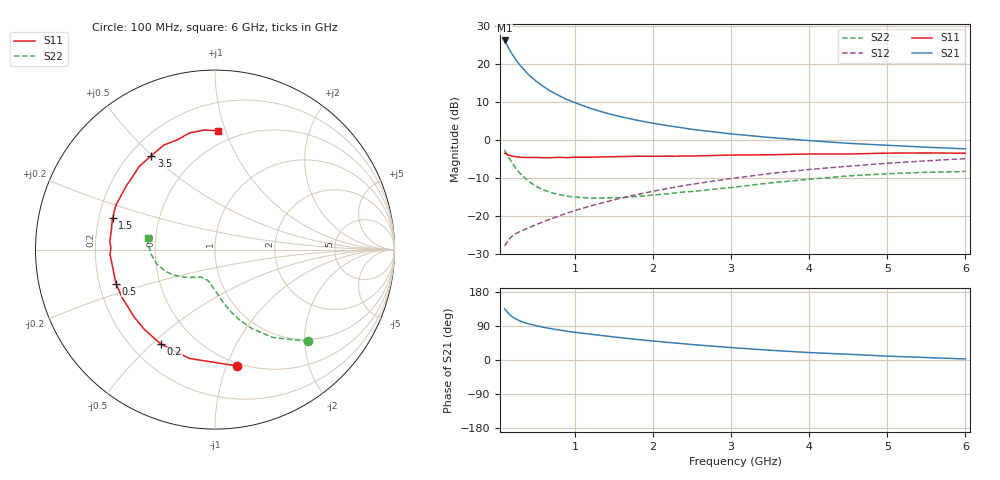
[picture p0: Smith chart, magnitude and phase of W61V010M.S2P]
! SIEMENS Small Signal Semiconductors
! BFR193W
! Si NPN RF Bipolar Junction Transistor in SOT323
! VCE = 1 V  IC = 10 mA
! Common Emitter S-Parameters:  September  1992
# GHz  S  MA  R  50
!  f  S11  S21  S12  S22
! GHz  MAG  ANG  MAG  ANG  MAG  ANG  MAG  ANG
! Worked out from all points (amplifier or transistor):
!   28 points, 100 MHz to 6 GHz, reference 50 ohm
!   highest |S21| = 26.1 dB at 100 MHz (marker M1)
!   |S21| within 3 dB of that: start of sweep to 179.9 MHz
!   unconditionally stable (mu >= 1): 892.4 MHz to 2.755 GHz
!   at 300 MHz: K = 0.57, MSG = 21.8 dB, |S12| = -24.1 dB
!   at 1.5 GHz: K = 1.06, MAG = 9.6 dB, |S12| = -15.8 dB
!   at 6 GHz: K = 0.95, MSG = 1.3 dB, |S12| = -5.0 dB
!   S11 on the Smith chart (normalised r, x): 100 MHz: 0.47, -1.09; 200 MHz: 0.32, -0.54; 500 MHz: 0.27, -0.15; 1.5 GHz: 0.26, +0.14; 3.5 GHz: 0.28, +0.50; 6 GHz: 0.40, +0.94
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0.1  0.6596 -79.3  20.18 135.3  0.0397 56.4  0.7291 -44.5
0.15  0.623 -103.2  16.11 122.6  0.0484 49.7  0.5863 -56.6
0.2  0.6067 -119.7  13.18 113.8  0.0542 46.5  0.4854 -65.0
0.25  0.5937 -131.6  11.02 107.7  0.0585 45.4  0.4094 -71.2
0.3  0.5867 -140.0  9.453 102.9  0.0622 45.5  0.3584 -75.6
0.4  0.5827 -152.8  7.275 95.8  0.0687 46.9  0.2868 -82.3
0.5  0.5831 -161.1  5.913 90.7  0.0759 49.3  0.2441 -87.2
0.6  0.5785 -167.7  4.975 86.3  0.0836 51.2  0.2178 -91.9
0.7  0.5798 -172.8  4.277 82.5  0.0913 53.1  0.2005 -95.2
0.8  0.5856 -177.3  3.775 79.1  0.0993 54.8  0.1895 -98.6
0.9  0.5798 179.0  3.37 76.0  0.108 56.2  0.1805 -101.1
1  0.588 175.5  3.064 73.1  0.1166 57.4  0.176 -103.7
1.2  0.5875 169.4  2.579 68.1  0.1343 58.8  0.1701 -109.4
1.5  0.5966 162.6  2.106 60.8  0.1614 60.0  0.1722 -115.9
1.8  0.6055 155.5  1.796 54.2  0.1902 60.0  0.179 -121.5
2.2  0.6055 146.9  1.521 46.3  0.2292 59.1  0.1945 -127.5
2.5  0.6097 141.2  1.366 40.8  0.259 57.8  0.2083 -132.0
3  0.6269 132.3  1.191 32.8  0.3085 54.8  0.2347 -139.5
3.5  0.6326 124.1  1.067 25.7  0.3587 50.9  0.2697 -148.0
4.5  0.647 108.7  0.896 15.2  0.4472 42.3  0.3337 -166.1
5.5  0.6689 95.3  0.796 6.5  0.5266 33.3  0.372 176.1
6  0.6624 88.6  0.757 2.8  0.5625 28.5  0.3813 170.3
